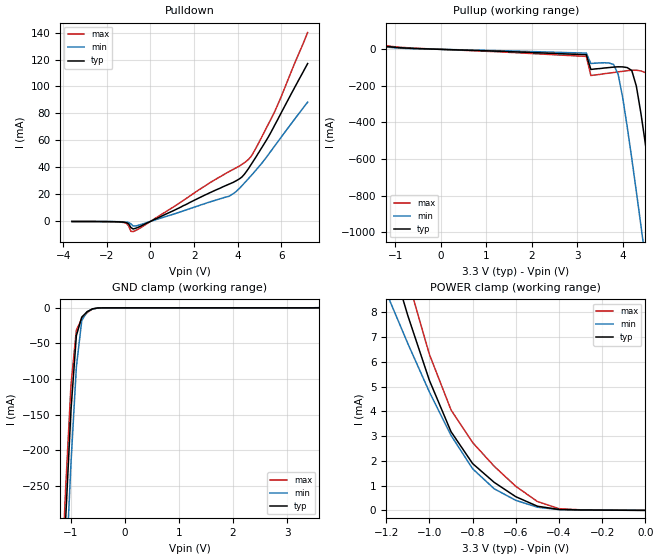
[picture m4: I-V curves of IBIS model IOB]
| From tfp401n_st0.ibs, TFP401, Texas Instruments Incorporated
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|   INPUT / OUTPUT  MODEL
[Model]   IOB
Model_type   I/O
Vinl = 0.8
Vinh = 2.0
| variable   typ   min   max
C_comp   2pF   NA   NA
|   typ   min   max
[Temperature Range]   25.0   70   0
[Voltage range]   3.3V   3.0V   3.6V
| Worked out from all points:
|   slope of the pulldown table from 0 to 0.495 V, typ, clamps not added: 130 ohm
|   slope of the pullup table from 0 to 0.495 V, typ, clamps not added: 124 ohm
|   GND clamp passes 1 mA (typ) near -0.57 V on its own axis
|   POWER clamp passes 1 mA (typ) near -0.68 V on its own axis
[GND_clamp]
|Voltage   I(typ)   I(min)   I(max)
-3.6V     -5.15A     -5.23A     -5.11A
-1.2V     -475mA     -560mA     -430mA
-1.1V     -300mA     -383mA     -257mA
-1V       -144mA     -219mA     -109mA
-900mV    -39.2mA    -83.2mA    -31.5mA
-800mV    -13mA      -17.8mA    -15.2mA
-700mV    -5.45mA    -5.42mA    -6.6mA
-600mV    -1.39mA    -1.57mA    -1.6mA
-400mV    -9.37uA    -21uA      -7.8uA
3.6V      15.8uA     404uA      155pA
[Power_clamp]
|Note that the [Power_clamp] voltage table is referenced to Vcc
|and is calculated using Vtable=Vcc-Vmeasured.
|Voltage   I(typ)   I(min)   I(max)
-3.3V     79.9mA     56.2mA     103mA
-1.2V     10.8mA     8.81mA     12.9mA
-1.1V     7.87mA     6.74mA     9.33mA
-1V       5.25mA     4.78mA     6.3mA
-900mV    3.18mA     3.03mA     4.06mA
-800mV    1.89mA     1.68mA     2.74mA
-700mV    1.13mA     871uA      1.78mA
-600mV    551uA      404uA      970uA
-500mV    167uA      127uA      357uA
-400mV    34.7uA     29.7uA     68.4uA
-300mV    15.8uA     12.9uA     20.6uA
0V        146pA      221pA      155pA
[Pulldown]
|Voltage   I(typ)   I(min)   I(max)
-3.6V     -61.5uA    -42.8uA    -79.1uA
-1.3V     -473uA     -291uA     -661uA
-1.1V     -994uA     -538uA     -1.54mA
-1V       -1.9mA     -876uA     -3.36mA
-900mV    -4.47mA    -1.78mA    -7.33mA
-800mV    -5.66mA    -3.31mA    -7.6mA
3.6V      27.6mA     18.6mA     36.9mA
4.1V      31.8mA     24.9mA     41.3mA
4.4V      37.1mA     30.1mA     44.7mA
4.7V      44.4mA     35.5mA     50.5mA
5.7V      71.6mA     56.1mA     81.7mA
7.2V      117mA      88.4mA     140mA
[Pullup]
|Note that the [Pullup] voltage table is referenced to Vcc
|and is calculated using Vtable=Vcc-Vmeasured.
|Voltage   I(typ)   I(min)   I(max)
-3.3V     81.7mA     57.7mA     106mA
3.2V      -29.3mA    -20.5mA    -38.6mA
3.3V      -110mA     -77.4mA    -143mA
3.8V      -97.2mA    -82.8mA    -127mA
4V        -96mA      -264mA     -120mA
4.2V      -116mA     -598mA     -114mA
4.4V      -349mA     -962mA     -118mA
4.5V      -519mA     -1.15A     -127mA
4.6V      -697mA     -1.34A     -177mA
4.8V      -1.07A     -1.72A     -474mA
5.1V      -1.63A     -2.29A     -1.02A
6.6V      -4.56A     -5.23A     -3.92A
[Ramp]
|   typ   min   max
dV/dt_r   2.03v/1.1ns   1.82v/1.7ns   1.93v/600ps
dV/dt_f   1.98v/900ps   1.80v/1.5ns   2.22v/600ps
R_load = 5K
